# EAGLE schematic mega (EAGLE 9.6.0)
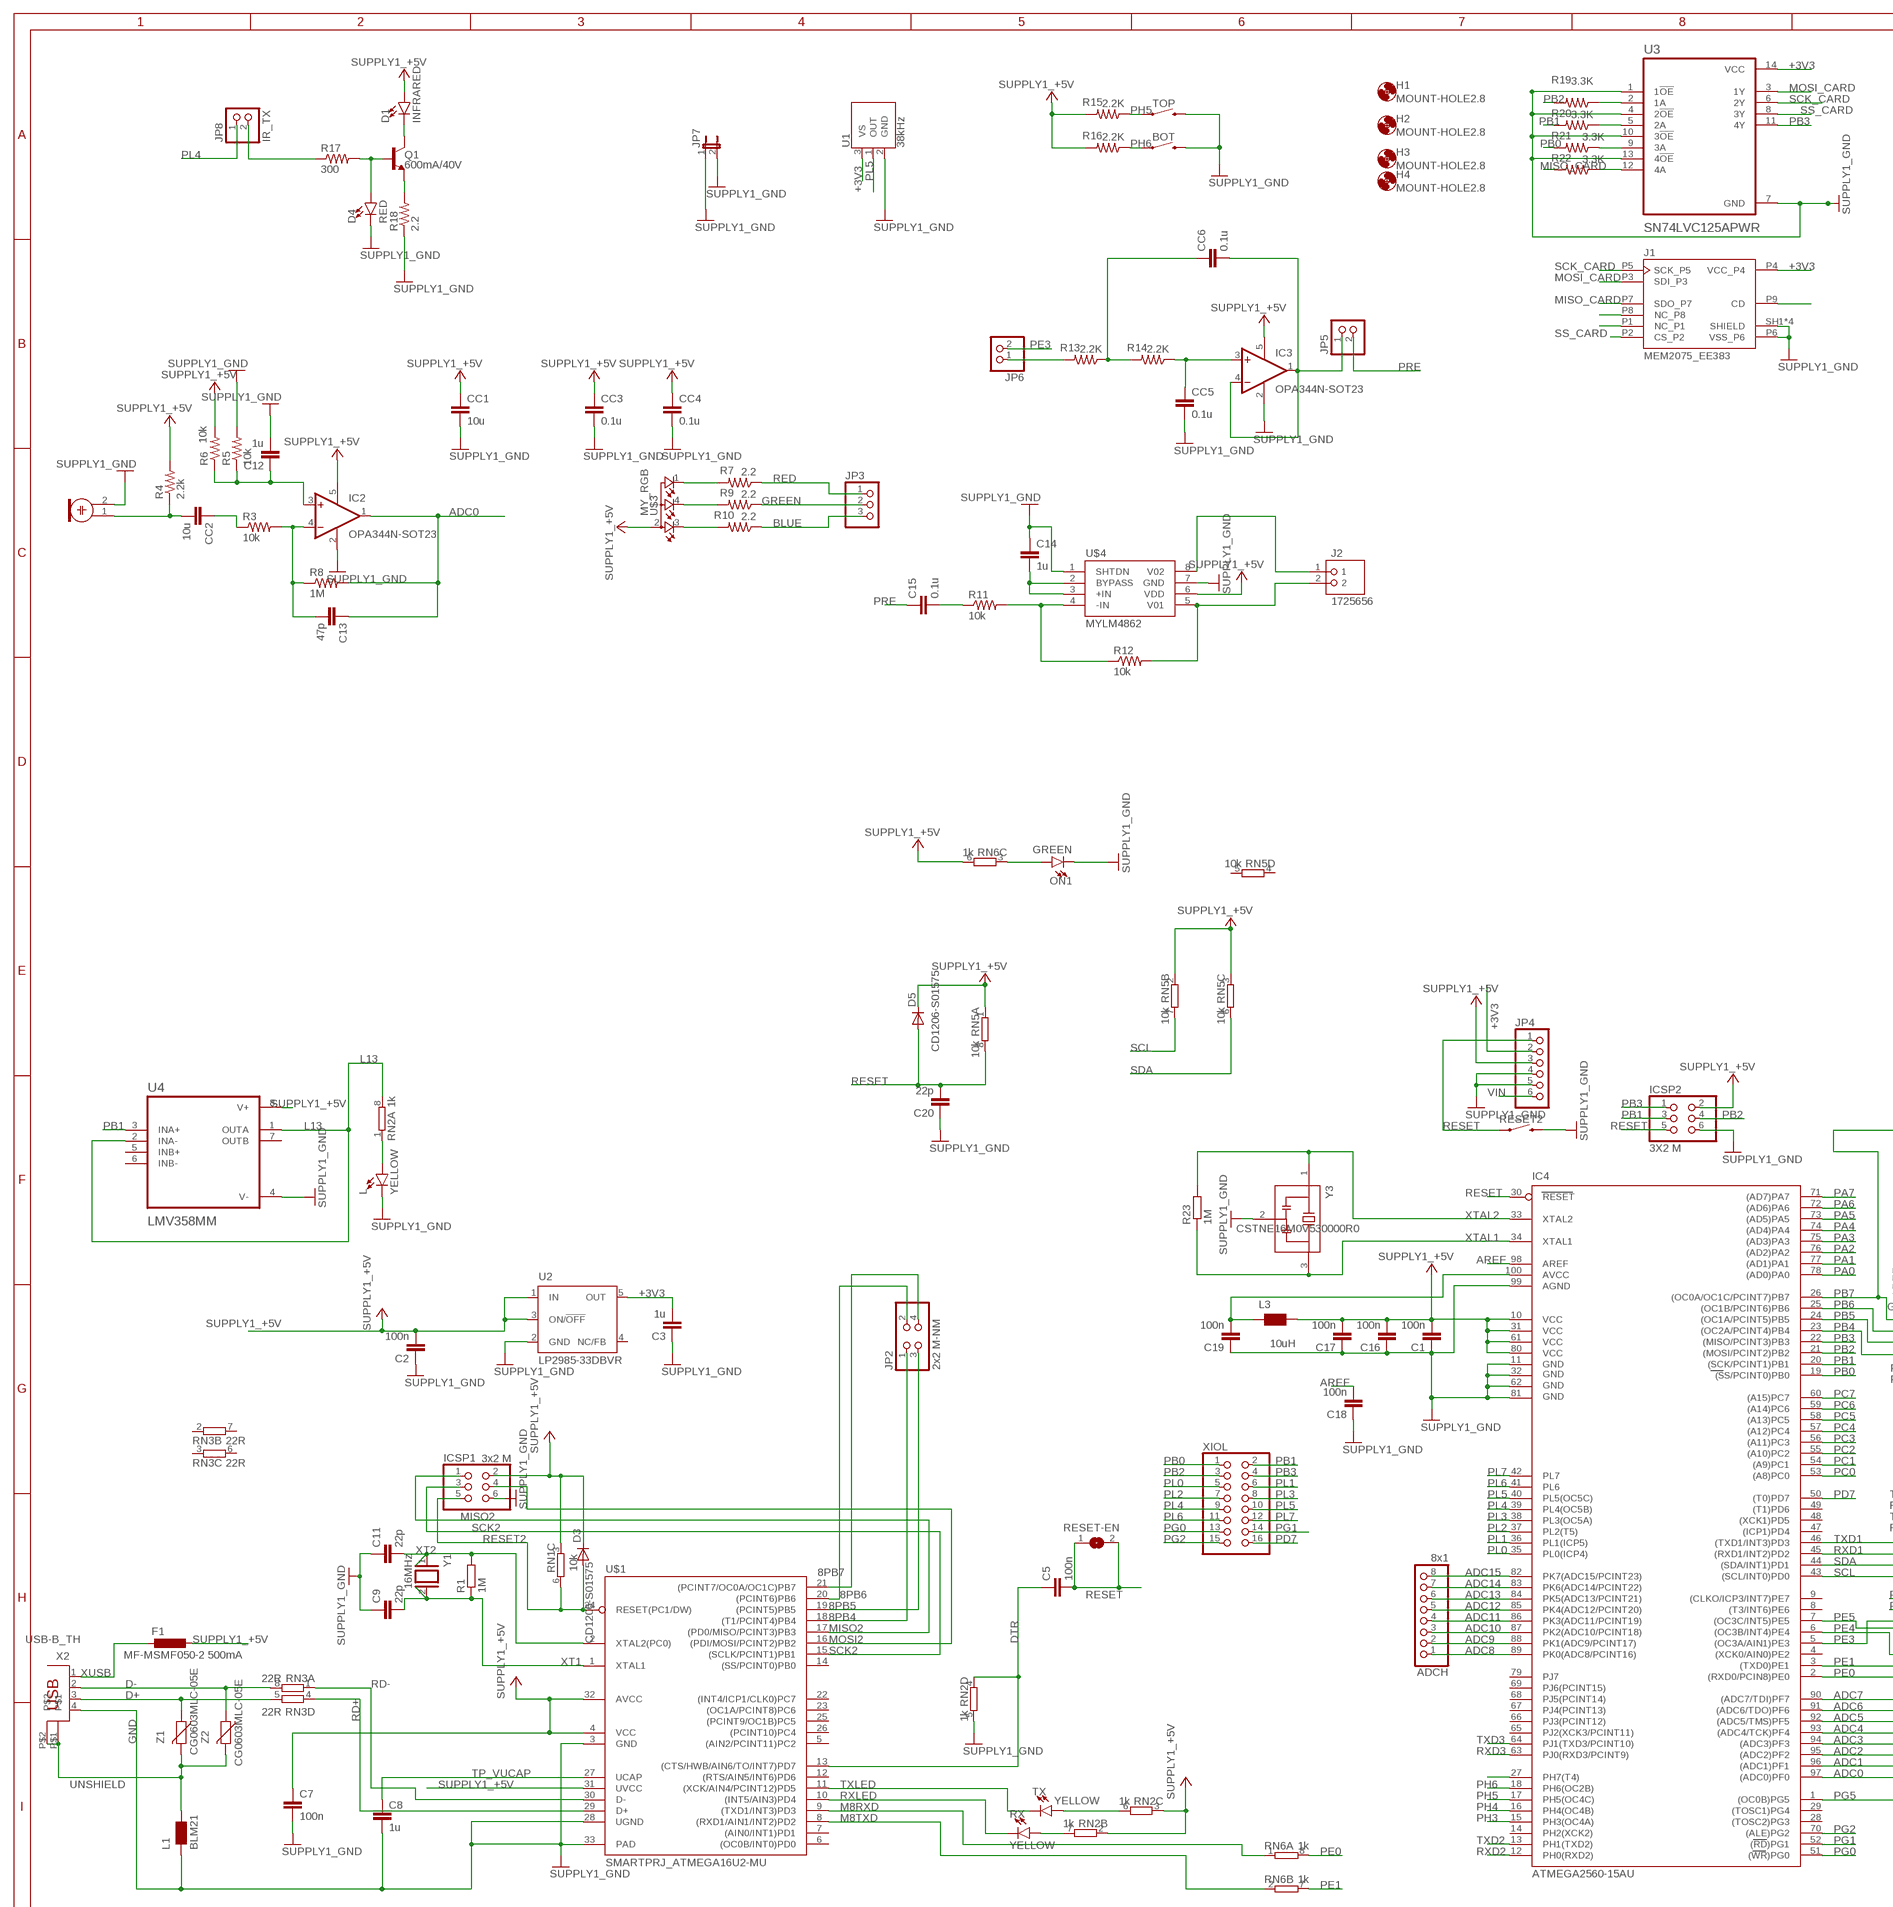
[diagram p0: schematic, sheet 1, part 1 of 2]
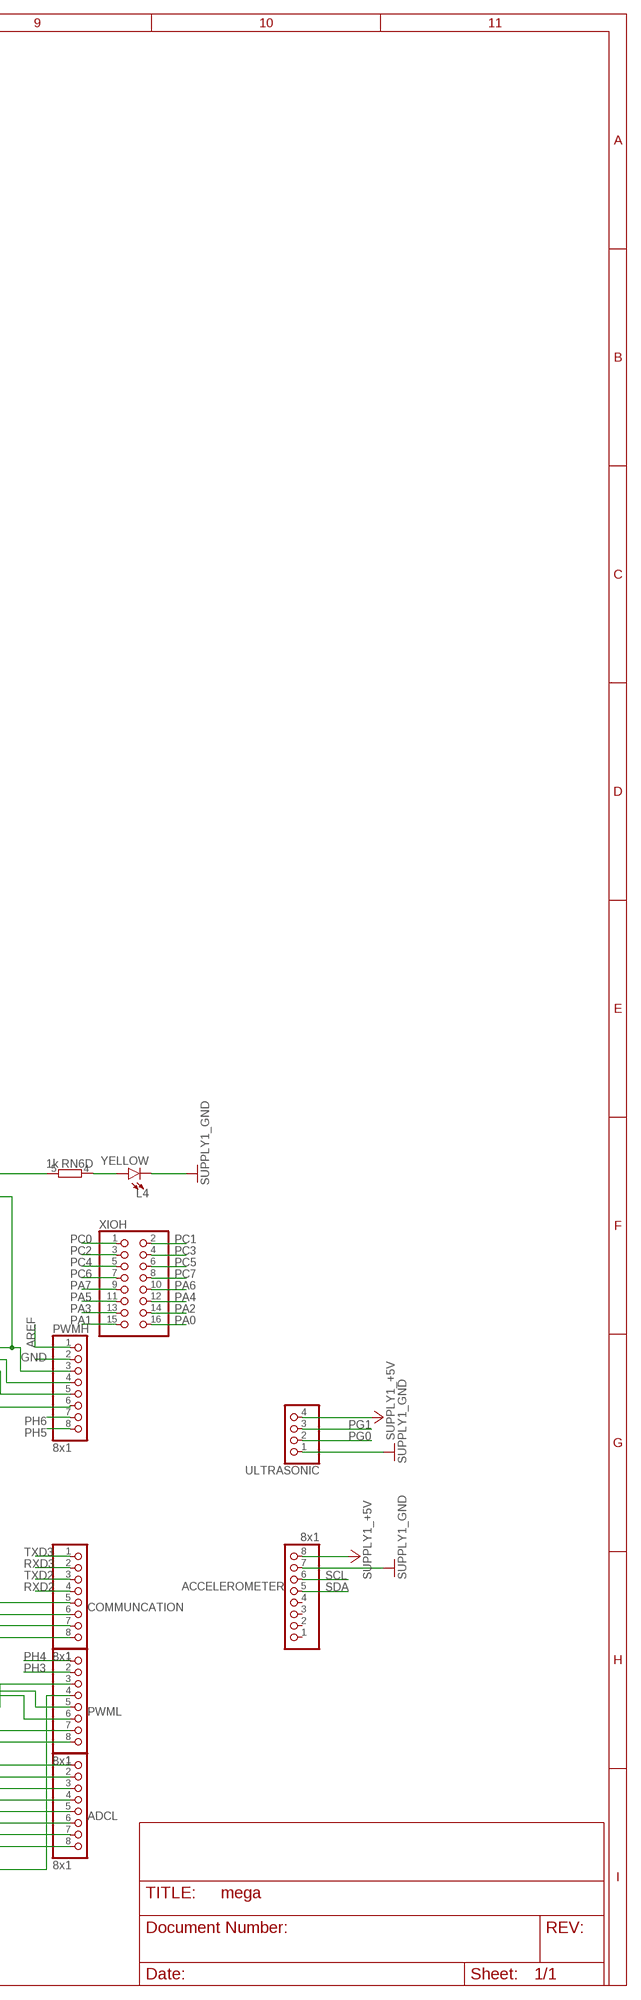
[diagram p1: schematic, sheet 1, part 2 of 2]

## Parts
ACCELEROMETER  8x1  SMARTPRJ_PINHD-1X8  [SMARTPRJ_1X08]
ADCH  8x1  SMARTPRJ_PINHD-1X8  [SMARTPRJ_1X08]
ADCL  8x1  SMARTPRJ_PINHD-1X8  [SMARTPRJ_1X08]
BOT  MOMENTARY-SWITCH-SPST-SMD-5.2-REDUNDANT  [TACTILE_SWITCH_SMD_5.2MM]
C1  100n  SMARTPRJ_C-EUC1206  [SMARTPRJ_C1206]
C2  100n  SMARTPRJ_C-EUC1206  [SMARTPRJ_C1206]
C3  1u  SMARTPRJ_C-EUC1206  [SMARTPRJ_C1206]
C5  100n  SMARTPRJ_C-EUC1206  [SMARTPRJ_C1206]
C7  100n  SMARTPRJ_C-EUC1206  [SMARTPRJ_C1206]
C8  1u  SMARTPRJ_C-EUC1206  [SMARTPRJ_C1206]
C9  22p  SMARTPRJ_C-EUC1206  [SMARTPRJ_C1206]
C11  22p  SMARTPRJ_C-EUC1206  [SMARTPRJ_C1206]
C12  1u  SMARTPRJ_C-EUC1206  [SMARTPRJ_C1206]
C13  47p  SMARTPRJ_C-EUC1206  [SMARTPRJ_C1206]
C14  1u  SMARTPRJ_C-EUC1206  [SMARTPRJ_C1206]
C15  0.1u  SMARTPRJ_C-EUC1206  [SMARTPRJ_C1206]
C16  100n  SMARTPRJ_C-EUC1206  [SMARTPRJ_C1206]
C17  100n  SMARTPRJ_C-EUC1206  [SMARTPRJ_C1206]
C18  100n  SMARTPRJ_C-EUC1206  [SMARTPRJ_C1206]
C19  100n  SMARTPRJ_C-EUC1206  [SMARTPRJ_C1206]
C20  22p  SMARTPRJ_C-EUC1206  [SMARTPRJ_C1206]
CC1  10u  SMARTPRJ_C-EUC1206  [SMARTPRJ_C1206]
CC2  10u  SMARTPRJ_C-EUC1206  [SMARTPRJ_C1206]
CC3  0.1u  SMARTPRJ_C-EUC1206  [SMARTPRJ_C1206]
CC4  0.1u  SMARTPRJ_C-EUC1206  [SMARTPRJ_C1206]
CC5  0.1u  SMARTPRJ_C-EUC1206  [SMARTPRJ_C1206]
CC6  0.1u  SMARTPRJ_C-EUC1206  [SMARTPRJ_C1206]
COMMUNCATION  8x1  SMARTPRJ_PINHD-1X8  [SMARTPRJ_1X08]
D1  INFRARED  LED1206  [LED-1206]
D3  CD1206-S01575  DIODE_DIODE-MINIMELF  [DIODE_MINIMELF]
D4  RED  LED1206  [LED-1206]
D5  CD1206-S01575  DIODE_DIODE-MINIMELF  [DIODE_MINIMELF]
F1  MF-MSMF050-2 500mA  RCL_L-EUL1812  [RCL_L1812]
H1  MOUNT-HOLE2.8  [2,8]
H2  MOUNT-HOLE2.8  [2,8]
H3  MOUNT-HOLE2.8  [2,8]
H4  MOUNT-HOLE2.8  [2,8]
IC2  OPA344N-SOT23  [SOT23-5]
IC3  OPA344N-SOT23  [SOT23-5]
IC4  ATMEGA2560-15AU  INTEGRATEDCIRCUITS_0023_ATMEGA2560-16AU  [INTEGRATEDCIRCUITS_TQFP100]
ICSP1  3x2 M  PINHD-2X3  [2X03]
ICSP2  3X2 M  SMARTPRJ_PINHD-2X3  [SMARTPRJ_2X03]
J1  MEM2075_EE383  [GCT_MEM2075-00-140-01-A]
J2  1725656  [PHOENIX_1725656]
JP2  2x2 M-NM  SMARTPRJ_PINHD-2X2  [SMARTPRJ_2X02]
JP3  PINHD-1X3  [1X03]
JP4  PINHD-1X6  [1X06]
JP5  PINHD-1X2  [1X02]
JP6  PINHD-1X2  [1X02]
JP7  JP1E  [JP1]
JP8  IR_TX  PINHD-1X2  [1X02]
L  YELLOW  LED1206  [LED-1206]
L1  BLM21  WUERTH-ELEKTRONIK_WE-CBF_1206  [WUERTH-ELEKTRONIK_1206]
L3  10uH  INDUTTANZE_0715_CV201210-100K  [INDUTTANZE_0805]
L4  YELLOW  LED1206  [LED-1206]
ON1  GREEN  LED1206  [LED-1206]
PWMH  8x1  SMARTPRJ_PINHD-1X8  [SMARTPRJ_1X08]
PWML  8x1  SMARTPRJ_PINHD-1X8  [SMARTPRJ_1X08]
Q1  600mA/40V  TRANS_NPN-MMBT2222AL  [SOT23-3]
R1  1M  SMARTPRJ_R-EU_M1206  [SMARTPRJ_M1206]
R3  10k  R-US_R1206  [R1206]
R4  2.2k  R-US_R1206  [R1206]
R5  10k  R-US_R1206  [R1206]
R6  10k  R-US_R1206  [R1206]
R7  2.2  R-US_R1206  [R1206]
R8  1M  R-US_R1206  [R1206]
R9  2.2  R-US_R1206  [R1206]
R10  2.2  R-US_R1206  [R1206]
R11  10k  R-US_R1206  [R1206]
R12  10k  R-US_R1206  [R1206]
R13  2.2K  R-US_R1206  [R1206]
R14  2.2K  R-US_R1206  [R1206]
R15  2.2K  R-US_R1206  [R1206]
R16  2.2K  R-US_R1206  [R1206]
R17  300  R-US_R1206  [R1206]
R18  2.2  R-US_R1206  [R1206]
R19  3.3K  R-US_R1206  [R1206]
R20  3.3K  R-US_R1206  [R1206]
R21  3.3K  R-US_R1206  [R1206]
R22  3.3K  R-US_R1206  [R1206]
R23  1M  SMARTPRJ_R-EU_R1206  [SMARTPRJ_R1206]
RESET2  MOMENTARY-SWITCH-SPST-SMD-5.2-REDUNDANT  [TACTILE_SWITCH_SMD_5.2MM]
RESET-EN  JUMPER_SJ  [JUMPER_SJ]
RN1  10k  RESISTOR-DIL_4R-NCAY16  [RESISTOR-DIL_CAY16]
RN2  1k  RESISTOR-DIL_4R-NCAY16  [RESISTOR-DIL_CAY16]
RN3  22R  RESISTOR-DIL_4R-NCAY16  [RESISTOR-DIL_CAY16]
RN5  10k  RESISTOR-DIL_4R-NCAY16  [RESISTOR-DIL_CAY16]
RN6  1k  RESISTOR-DIL_4R-NCAY16  [RESISTOR-DIL_CAY16]
RX  YELLOW  LED1206  [LED-1206]
TOP  MOMENTARY-SWITCH-SPST-SMD-5.2-REDUNDANT  [TACTILE_SWITCH_SMD_5.2MM]
TX  YELLOW  LED1206  [LED-1206]
U1  38kHz  TSOP38238  [TSOP382]
U2  LP2985-33DBVR  SMARTPRJ_LP2985-XXDBVR33  [SMARTPRJ_SOT23-DBV]
U3  SN74LVC125APWR  [SOP65P640X120-14N]
U4  LMV358MM  [SOP65P490X110-8N]
U$1  SMARTPRJ_ATMEGA16U2-MU  [SMARTPRJ_MLF32]
U$2  PIC_MICROPHONE  [WM-62PC/62PK]
U$3  MY_RGB  [GM1WA55311A]
U$4  MYLM4862  [MYSOIC8]
ULTRASONIC  PINHD-1X4  [1X04]
X2  USB-B_TH  SMARTPRJ_PN61729  [SMARTPRJ_PN61729]
XIOH  PINHD-2X8  [2X08]
XIOL  PINHD-2X8  [2X08]
Y1  16MHz  SMARTPRJ_XTAL/S  [SMARTPRJ_QS]
Y3  CSTNE16M0V530000R0  [OSC_CSTNE16M0V530000R0]
Z1  CG0603MLC-05E  VARISTOR_VARISTORCN0603  [VARISTOR_CT/CN0603]
Z2  CG0603MLC-05E  VARISTOR_VARISTORCN0603  [VARISTOR_CT/CN0603]

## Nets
8PB4: JP2.1 U$1.18((T1/PCINT4)PB4)
8PB5: JP2.3 U$1.19((PCINT5)PB5)
8PB6: JP2.2 U$1.20((PCINT6)PB6)
8PB7: JP2.4 U$1.21((PCINT7/OC0A/OC1C)PB7)
+3V3: C3.2 J1.P4(VCC_P4) JP4.2 U1.3(VS) U2.5(OUT) U3.14(VCC)
ADC0: ADCL.8 C13.1 IC2.1(OUT) IC4.97((ADC0)PF0) R8.2
ADC1: ADCL.7 IC4.96((ADC1)PF1)
ADC2: ADCL.6 IC4.95((ADC2)PF2)
ADC3: ADCL.5 IC4.94((ADC3)PF3)
ADC4: ADCL.4 IC4.93((ADC4/TCK)PF4)
ADC5: ADCL.3 IC4.92((ADC5/TMS)PF5)
ADC6: ADCL.2 IC4.91((ADC6/TDO)PF6)
ADC7: ADCL.1 IC4.90((ADC7/TDI)PF7)
ADC8: ADCH.1 IC4.89(PK0(ADC8/PCINT16))
ADC9: ADCH.2 IC4.88(PK1(ADC9/PCINT17))
ADC10: ADCH.3 IC4.87(PK2(ADC10/PCINT18))
ADC11: ADCH.4 IC4.86(PK3(ADC11/PCINT19))
ADC12: ADCH.5 IC4.85(PK4(ADC12/PCINT20))
ADC13: ADCH.6 IC4.84(PK5(ADC13/PCINT21))
ADC14: ADCH.7 IC4.83(PK6(ADC14/PCINT22))
ADC15: ADCH.8 IC4.82(PK7(ADC15/PCINT23))
AREF: C18.2 IC4.98(AREF) PWMH.1
BLUE: JP3.3 R10.1
D+: RN3.5 X2.3 Z1.1
D-: RN3.8 X2.2 Z2.1
DTR: C5.1 RN2.4 U$1.13((CTS/HWB/AIN6/TO/INT7)PD7)
GND: ACCELEROMETER.7 BOT.3 BOT.4 C1.1 C2.1 C3.1 C7.2 C8.2 C9.1 C11.1 C12.2 C14.1 C16.1 C17.1 C18.1 C19.1 C20.1 CC1.2 CC3.2 CC4.2 CC5.2 D4.C IC2.2(V-) IC3.2(V-) IC4.11(GND) IC4.32(GND1) IC4.62(GND2) IC4.81(GND3) IC4.99(AGND) ICSP1.6 ICSP2.6 J1.P6(VSS_P6) J1.SH1(SHIELD) J1.SH2(SHIELD) J1.SH3(SHIELD) J1.SH4(SHIELD) JP4.4 JP4.5 JP7.1 JP7.2 L1.1 L4.C L.C ON1.C PWMH.2 R5.2 R18.1 RESET2.3 RESET2.4 RN2.5 TOP.3 TOP.4 U1.2(GND) U2.2(GND) U3.1(1!OE) U3.4(2!OE) U3.7(GND) U3.10(3!OE) U3.13(4!OE) U4.4(V-) U$1.3(GND) U$1.28(UGND) U$1.33(PAD) U$2.2 U$4.1(SHTDN) U$4.7(GND) ULTRASONIC.1 X2.4 Y3.2(GND) ; supply symbol labelled SUPPLY1_GND
GREEN: JP3.2 R9.1
L13: RN2.8 U4.1(OUTA) U4.2(INA-)
M8RXD: RN6.1 U$1.9((TXD1/INT3)PD3)
M8TXD: RN6.2 U$1.8((RXD1/AIN1/INT2)PD2)
MISO2: ICSP1.1 U$1.17((PD0/MISO/PCINT3)PB3)
MISO_CARD: J1.P7(SDO_P7) R22.2
MOSI2: ICSP1.4 U$1.16((PDI/MOSI/PCINT2)PB2)
MOSI_CARD: J1.P3(SDI_P3) U3.3(1Y)
N$1: CC6.1 R13.1 R14.2
N$2: RN2.7 RX.A
N$3: C12.1 IC2.3(+IN) R5.1 R6.1
N$4: RN2.6 TX.A
N$6: R10.2 U$3.3
N$7: C13.2 IC2.4(-IN) R3.2 R8.1
N$8: L.A RN2.1
N$9: ON1.A RN6.3
N$10: CC2.1 R3.1
N$11: CC2.2 R4.1 U$2.1
N$12: R9.2 U$3.4
N$13: R7.2 U$3.1
N$14: C14.2 U$4.2(BYPASS) U$4.3(+IN)
N$15: R11.2 R12.1 U$4.4(-IN)
N$16: C15.2 R11.1
N$17: J2.2 R12.2 U$4.5(V01)
N$18: J2.1 U$4.8(V02)
N$19: JP6.1 R13.2
N$20: CC5.1 IC3.3(+IN) R14.1
N$21: CC6.2 IC3.1(OUT) IC3.4(-IN) JP5.1
N$22: J1.P8(NC_P8)
N$23: J1.P1(NC_P1)
N$24: C19.2 IC4.100(AVCC) L3.1
N$25: J1.P9(CD)
N$26: L4.A RN6.4
N$27: JP8.2 R17.1
N$28: D4.A Q1.1(B) R17.2
N$29: Q1.2(E) R18.2
N$30: D1.C Q1.3(C)
N$33: R21.1 U3.9(3A)
N$34: R20.1 U3.5(2A)
N$35: R19.1 U3.2(1A)
N$36: R22.1 U3.12(4A)
N$124: IC4.27(PH7(T4))
PA0: IC4.78((AD0)PA0) XIOH.16
PA1: IC4.77((AD1)PA1) XIOH.15
PA2: IC4.76((AD2)PA2) XIOH.14
PA3: IC4.75((AD3)PA3) XIOH.13
PA4: IC4.74((AD4)PA4) XIOH.12
PA5: IC4.73((AD5)PA5) XIOH.11
PA6: IC4.72((AD6)PA6) XIOH.10
PA7: IC4.71((AD7)PA7) XIOH.9
PB0: IC4.19((SS/PCINT0)PB0) R21.2 XIOL.1
PB1: IC4.20((SCK/PCINT1)PB1) ICSP2.3 R20.2 U4.3(INA+) XIOL.2
PB2: IC4.21((MOSI/PCINT2)PB2) ICSP2.4 R19.2 XIOL.3
PB3: IC4.22((MISO/PCINT3)PB3) ICSP2.1 U3.11(4Y) XIOL.4
PB4: IC4.23((OC2A/PCINT4)PB4) PWMH.6
PB5: IC4.24((OC1A/PCINT5)PB5) PWMH.5
PB6: IC4.25((OC1B/PCINT6)PB6) PWMH.4
PB7: IC4.26((OC0A/OC1C/PCINT7)PB7) PWMH.3 RN6.5
PC0: IC4.53((A8)PC0) XIOH.1
PC1: IC4.54((A9)PC1) XIOH.2
PC2: IC4.55((A10)PC2) XIOH.3
PC3: IC4.56((A11)PC3) XIOH.4
PC4: IC4.57((A12)PC4) XIOH.5
PC5: IC4.58((A13)PC5) XIOH.6
PC6: IC4.59((A14)PC6) XIOH.7
PC7: IC4.60((A15)PC7) XIOH.8
PD7: IC4.50((T0)PD7) XIOL.16
PE0: IC4.2((RXD0/PCIN8)PE0) PWML.8 RN6.8
PE1: IC4.3((TXD0)PE1) PWML.7 RN6.7
PE3: IC4.5((OC3A/AIN1)PE3) JP6.2 PWML.3
PE4: IC4.6((OC3B/INT4)PE4) PWML.6
PE5: IC4.7((OC3C/INT5)PE5) PWML.5
PG0: IC4.51((WR)PG0) ULTRASONIC.2 XIOL.13
PG1: IC4.52((RD)PG1) ULTRASONIC.3 XIOL.14
PG2: IC4.70((ALE)PG2) XIOL.15
PG5: IC4.1((OC0B)PG5) PWML.4
PH3: IC4.15(PH3(OC4A)) PWML.2
PH4: IC4.16(PH4(OC4B)) PWML.1
PH5: IC4.17(PH5(OC4C)) PWMH.8 R15.1 TOP.1 TOP.2
PH6: BOT.1 BOT.2 IC4.18(PH6(OC2B)) PWMH.7 R16.1
PL0: IC4.35(PL0(ICP4)) XIOL.5
PL1: IC4.36(PL1(ICP5)) XIOL.6
PL2: IC4.37(PL2(T5)) XIOL.7
PL3: IC4.38(PL3(OC5A)) XIOL.8
PL4: IC4.39(PL4(OC5B)) JP8.1 XIOL.9
PL5: IC4.40(PL5(OC5C)) U1.1(OUT) XIOL.10
PL6: IC4.41(PL6) XIOL.11
PL7: IC4.42(PL7) XIOL.12
PRE: C15.1 JP5.2
RD+: RN3.4 U$1.29(D+)
RD-: RN3.1 U$1.30(D-)
RED: JP3.1 R7.1
RESET: C5.2 C20.2 D5.A IC4.30(RESET) ICSP2.5 JP4.1 RESET2.1 RESET2.2 RESET-EN.1 RESET-EN.2 RN5.8
RESET2: D3.A ICSP1.5 RN1.6 U$1.24(RESET(PC1/DW))
RXD1: COMMUNCATION.6 IC4.45((RXD1/INT2)PD2)
RXD2: COMMUNCATION.4 IC4.12(PH0(RXD2))
RXD3: COMMUNCATION.2 IC4.63(PJ0(RXD3/PCINT9))
RXLED: RX.C U$1.10((INT5/AIN3)PD4)
SCK2: ICSP1.3 U$1.15((SCLK/PCINT1)PB1)
SCK_CARD: J1.P5(SCK_P5) U3.6(2Y)
SCL: ACCELEROMETER.6 COMMUNCATION.8 IC4.43((SCL/INT0)PD0) RN5.7
SDA: ACCELEROMETER.5 COMMUNCATION.7 IC4.44((SDA/INT1)PD1) RN5.6
SS_CARD: J1.P2(CS_P2) U3.8(3Y)
SUPPLY1_+5V: ACCELEROMETER.8 C1.2 C2.2 C7.1 C16.2 C17.2 CC1.1 CC3.1 CC4.1 D1.A D3.C D5.C F1.2 IC2.5(V+) IC3.5(V+) IC4.10(VCC) IC4.31(VCC1) IC4.61(VCC2) IC4.80(VCC3) ICSP1.2 ICSP2.2 JP4.3 L3.2 R4.2 R6.2 R15.2 R16.2 RN1.3 RN2.2 RN2.3 RN5.1 RN5.2 RN5.3 RN6.6 U2.1(IN) U2.3(ON/!OFF) U4.8(V+) U$1.4(VCC) U$1.31(UVCC) U$1.32(AVCC) U$3.2 U$4.6(VDD) ULTRASONIC.4
TP_VUCAP: C8.1 U$1.27(UCAP)
TXD1: COMMUNCATION.5 IC4.46((TXD1/INT3)PD3)
TXD2: COMMUNCATION.3 IC4.13(PH1(TXD2))
TXD3: COMMUNCATION.1 IC4.64(PJ1(TXD3/PCINT10))
TXLED: TX.C U$1.11((XCK/AIN4/PCINT12)PD5)
UNSHIELD: L1.2 X2.P$1 X2.P$2 Z1.2 Z2.2
VIN: JP4.6
XT1: C9.2 R1.1 U$1.1(XTAL1) Y1.2
XT2: C11.2 R1.2 U$1.2(XTAL2(PC0)) Y1.1
XTAL1: IC4.34(XTAL1) R23.1 Y3.3(OUT)
XTAL2: IC4.33(XTAL2) R23.2 Y3.1(IN)
XUSB: F1.1 X2.1
Unconnected: ACCELEROMETER.1 ACCELEROMETER.2 ACCELEROMETER.3 ACCELEROMETER.4 IC4.4((XCK0/AIN0)PE2) IC4.8((T3/INT6)PE6) IC4.9((CLKO/ICP3/INT7)PE7) IC4.14(PH2(XCK2)) IC4.28((TOSC2)PG3) IC4.29((TOSC1)PG4) IC4.47((ICP1)PD4) IC4.48((XCK1)PD5) IC4.49((T1)PD6) IC4.65(PJ2(XCK3/PCINT11)) IC4.66(PJ3(PCINT12)) IC4.67(PJ4(PCINT13)) IC4.68(PJ5(PCINT14)) IC4.69(PJ6(PCINT15)) IC4.79(PJ7) RN1.1 RN1.2 RN1.4 RN1.5 RN1.7 RN1.8 RN3.2 RN3.3 RN3.6 RN3.7 RN5.4 RN5.5 U2.4(NC/FB) U4.5(INB+) U4.6(INB-) U4.7(OUTB) U$1.5((AIN2/PCINT11)PC2) U$1.6((OC0B/INT0)PD0) U$1.7((AIN0/INT1)PD1) U$1.12((RTS/AIN5/INT6)PD6) U$1.14((SS/PCINT0)PB0) U$1.22((INT4/ICP1/CLK0)PC7) U$1.23((OC1A/PCINT8)PC6) U$1.25((PCINT9/OC1B)PC5) U$1.26((PCINT10)PC4)

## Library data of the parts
ACCELEROMETER ADCH ADCL COMMUNCATION PWMH PWML = UNO-TH_Rev3e:SMARTPRJ_PINHD-1X8: PIN HEADER
BOT RESET2 TOP = SparkFun-Switches:MOMENTARY-SWITCH-SPST: Momentary Switch (Pushbutton) - SPST; PROD_ID: SWCH-08247; SF_SKU: COM-08720
C1-C3 C5 C7-C9 C11-C20 CC1-CC6 = UNO-TH_Rev3e:SMARTPRJ_C-EU: CAPACITOR, European symbol
D1 D4 L L4 ON1 RX TX = SparkFun-LED:LED: LED (Generic)
D3 D5 = UNO-TH_Rev3e:DIODE_DIODE-: DIODE
F1 = UNO-TH_Rev3e:RCL_L-EU: INDUCTOR, European symbol
H1-H4 = holes:MOUNT-HOLE: MOUNTING HOLE with drill center marker
IC2 IC3 = linear:OPA*-SOT23: Single Operational Amplifier Low Power, Single-Supply, Rail-To-Rail Operational Amplifier Source: http://focus.ti.com/lit/ds/symlink/opa2345.pdf
IC4 = MEGA2560_Rev3e:INTEGRATEDCIRCUITS_0023_ATMEGA2560-16AU: 8-bit Microcontroller with 256K Bytes In-System Programmable Flash - ATMEGA2560-16AU; CASE: TQFP100_14x14; MONTHLY_USAGE: _____; PART_NUMBER: ATMEGA2560-16AU; PRICE: _____; SUPPLIER: _____; TYPE: Circuito_Integrato
ICSP1 = SmartPrj:PINHD-2X3: PIN HEADER
ICSP2 = UNO-TH_Rev3e:SMARTPRJ_PINHD-2X3: PIN HEADER
J1 = MEM2075-00-140-01-A:MEM2075_EE383: Micro SD Memory Card Connector, 1.4mm Profile SMT, Push-Push, with Normally open Switch Check availability; AVAILABILITY: Not in stock; CHECK_PRICES: https://www.snapeda.com/parts/MEM2075-00-140-01-A/Global+Connector+Technology/view-part/?ref=eda; DESCRIPTION: 9 (8 + 1) Position Card Connector microSD Surface Mount, Right Angle Gold; MF: Global Connector Technology; MP: MEM2075-00-140-01-A; PACKAGE: None; PRICE: None; SNAPEDA_LINK: https://www.snapeda.com/parts/MEM2075-00-140-01-A/Global+Connector+Technology/view-part/?ref=snap
J2 = 1725656:1725656; MANUFACTURER: Phoenix Contact; MAXIMUM_PACKAGE_HEIGHT: 8.65mm; PARTREV: 03.03.2021; STANDARD: Manufacturer Recommendations
JP2 = UNO-TH_Rev3e:SMARTPRJ_PINHD-2X2: PIN HEADER
JP3 = pinhead:PINHD-1X3: PIN HEADER
JP4 = pinhead:PINHD-1X6: PIN HEADER
JP5 JP6 JP8 = pinhead:PINHD-1X2: PIN HEADER
JP7 = jumper:JP1E: JUMPER
L1 = UNO-TH_Rev3e:WUERTH-ELEKTRONIK_WE-CBF: SMD EMI Suppression Ferrite Beads
L3 = UNO-TH_Rev3e:INDUTTANZE_0715_CV201210-100K: 10uH 0805; CASE: 0805; MONTHLY_USAGE: _____; PART_NUMBER: CV201210-100K; PRICE: _____; SUPPLIER: _____; TYPE: Induttanze
Q1 = SparkFun-DiscreteSemi:TRANS_NPN: NPN transistor Current controlled devices typically used to amplify current or used as a switch. BC547 - COM-08928 (TO-92 45V 100mA) (1.Collector 2.Base 3.Emitter) 2N3904 - COM-00521 (TO-92 40V 200mA) (1.Emitter 2.Base 3.Collector) P2N2222A - COM-12852 (TO-92 40V 600mA) (1.Collector 2.Base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; PROD_ID: TRANS-08049
R1 R23 = UNO-TH_Rev3e:SMARTPRJ_R-EU_: RESISTOR, European symbol
R3-R22 = resistor_3rdPin_v20:R-US_: RESISTOR, American symbol
RESET-EN = UNO-TH_Rev3e:JUMPER_SJ: SMD solder JUMPER
RN1-RN3 RN5 RN6 = UNO-TH_Rev3e:RESISTOR-DIL_4R-N: Array Chip Resistor Source: RS Component / Phycomp
U1 = SparkFun-Sensors:TSOP382: Vishay Semiconductor TSOP32838 - 38kHz IR Receiver These products are miniaturized IR receiver modules for infrared remote control systems. A PIN diode and a preamplifier are assembled on a leadframe, the epoxy package contains an IR filter. The demodulated output signal can be directly connected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; PROD_ID: SEN-10266
U2 = UNO-TH_Rev3e:SMARTPRJ_LP2985-XXDBVR: ULTRALOW-POWER 50-mA LOW-DROPOUT LINEAR REGULATORS 50-mA Low-Dropout Regulator Source: http://focus.ti.com/lit/ds/symlink/tps77001.pdf
U3 = SN74LVC125APWR:SN74LVC125APWR
U4 = LMV358MM:LMV358MM
U$1 = UNO-TH_Rev3e:SMARTPRJ_ATMEGA16U2-
U$2 = MyD:PIC_MICROPHONE
U$3 = MyD:MY_RGB
U$4 = LM4862M_NOPB:MYLM4862
ULTRASONIC = pinhead:PINHD-1X4: PIN HEADER
X2 = UNO-TH_Rev3e:SMARTPRJ_PN61729: BERG USB connector
XIOH XIOL = pinhead:PINHD-2X8: PIN HEADER
Y1 = UNO-TH_Rev3e:SMARTPRJ_XTAL/S: CRYSTAL
Y3 = CSTNE16M0V530000R0:CSTNE16M0V530000R0; MANUFACTURER: Murata; MAXIMUM_PACKAGE_HEIGHT: 1mm; PARTREV: JGC42-8853B; STANDARD: Manufacturer Recomendations
Z1 Z2 = UNO-TH_Rev3e:VARISTOR_VARISTOR: VARISTOR

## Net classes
0 default: width 0.305 mm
